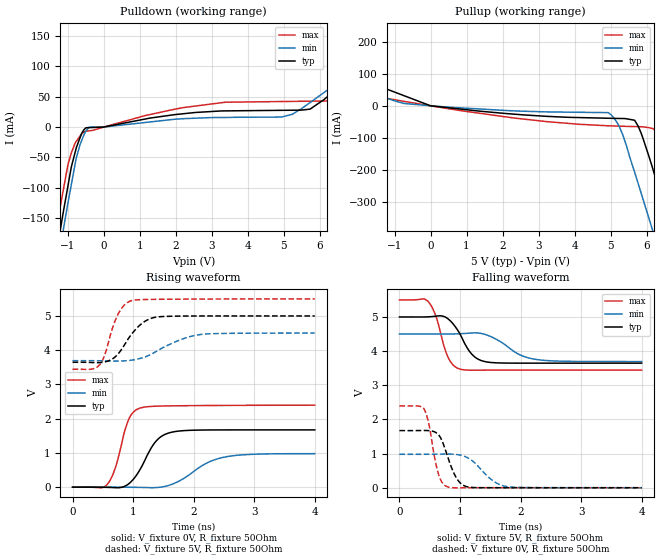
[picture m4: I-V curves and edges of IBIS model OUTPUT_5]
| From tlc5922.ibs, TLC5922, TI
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|   output_5 Model
[Model]   OUTPUT_5
Model_type   Output
Polarity   Non-Inverting
Vmeas = 2.5
Vref = 2.5
Cref = 15pF
Rref = 50
|   typ   min   max
|   (nom PVT)   (Fast PVT)   (slow PVT)
C_comp   1.655e-12   1.559e-12   1.779e-12
|ON state : BUFFER OUTPUT TURNED HIGH
|C_comp   1.655e-12   1.559e-12   1.779e-12
|OFF state: BUFFER OUTPUT TURNED LOW
|C_comp   1.494e-12   1.469e-12   1.521e-12
| Where nom  PVT is Nominal Process,  5V,  65C
|   Fast PVT is Strong Process,   5.5V,  -20C
|   Slow PVT is Weak Process,   4.5V,  125C
[Voltage Range]   5   4.5   5.5
|Ambient Temperature   25   85   -20
|Junction Temperature
[Temperature Range]   65   125   -20
[Pullup Reference]   5   4.5   5.5
[Pulldown Reference]   0   0   0
[Power Clamp Reference]   5   4.5   5.5
[GND Clamp Reference]   0   0   0
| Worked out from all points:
|   slope of the pulldown table from 0 to 0.75 V, typ, clamps not added: 87 ohm
|   slope of the pullup table from 0 to 0.75 V, typ, clamps not added: 81.5 ohm
|   falling waveform, V_fixture 5V, R_fixture 50Ohm: 20-80 % time 276ps typ, 433ps min, 206ps max; typ from 5 V to 3.65 V
|   rising waveform, V_fixture 0V, R_fixture 50Ohm: 20-80 % time 327ps typ, 542ps min, 224ps max; typ from 0 V to 1.67 V
|   rising waveform, V_fixture 5V, R_fixture 50Ohm: 20-80 % time 346ps typ, 567ps min, 233ps max; typ from 3.65 V to 5 V
|   falling waveform, V_fixture 0V, R_fixture 50Ohm: 20-80 % time 213ps typ, 343ps min, 153ps max; typ from 1.67 V to 0 V
[Pulldown]
|   Voltage   I(typ)   I(min)   I(max)
-5V       -1.603A    -1.604A    -1.595A
-1.305V   -205.4mA   -234.4mA   -164.9mA
-1.125V   -141.4mA   -171mA     -105mA
-990.5mV  -96.57mA   -124.8mA   -61.83mA
-755mV    -33.19mA   -49.9mA    -23.03mA
-391mV    -883.4uA   -118.5uA   -6.095mA
2.232V    22.09mA    13.87mA    32.24mA
5.233V    27.75mA    20.88mA    42.27mA
6.44V     61.19mA    70.61mA    47.93mA
8.107V    146.8mA    145mA      144.6mA
8.855V    186.3mA    179.5mA    191.6mA
10V       250.4mA    232.7mA    267.1mA
[Pullup]
|   Voltage   I(typ)   I(min)   I(max)
-5V       213.6mA    187.3mA    242.2mA
-1.188V   50.77mA    22.65mA    22.65mA
0V        0A         0A         0A
4.936V    -38.77mA   -21.32mA   -62.17mA
5.255V    -39.46mA   -67.54mA   -63.38mA
5.665V    -44.88mA   -205.3mA   -64.66mA
5.85V     -85.23mA   -271.8mA   -65.17mA
6.15V     -187.1mA   -380.7mA   -70.24mA
6.473V    -307.6mA   -499.4mA   -112.9mA
6.654V    -374.8mA   -566.2mA   -169mA
7.243V    -596.5mA   -784.5mA   -396mA
10V       -1.65A     -1.818A    -1.473A
[Ramp]
R_load = 50
|   typ   min   max
dV/dt_r   1.00336/3.2663e-10   0.587084/5.42378e-10   1.43592/2.23561e-10
dV/dt_f   0.811682/2.75881e-10   0.483611/4.32773e-10   1.23387/2.05834e-10
[Falling Waveform]
V_fixture = 5V
V_fixture_min = 4.5V
V_fixture_max = 5.5V
R_fixture = 50Ohm
|   Time   V(typ)   V(min)   V(max)
0s        5V         4.5V       5.5V
475ps     5.004V     4.5V       5.453V
600ps     5.023V     4.499V     5.038V
800ps     4.949V     4.5V       3.831V
975ps     4.576V     4.508V     3.487V
1.2ns     3.901V     4.531V     3.442V
1.45ns    3.681V     4.467V     3.443V
1.975ns   3.648V     3.905V     3.444V
2.225ns   3.647V     3.765V     3.444V
4ns       3.647V     3.694V     3.444V
[Rising Waveform]
V_fixture = 0V
V_fixture_min = 0V
V_fixture_max = 0V
R_fixture = 50Ohm
|   Time   V(typ)   V(min)   V(max)
0s        300.2pV    1.699nV    286.7pV
575ps     -6.312mV   794.4uV    84.58mV
700ps     -14.82mV   240.7uV    531.1mV
925ps     93.85mV    -3.088mV   1.972V
1.125ns   547.6mV    -7.671mV   2.316V
1.375ns   1.336V     -12.45mV   2.364V
1.65ns    1.609V     89.18mV    2.375V
2.2ns     1.669V     688mV      2.384V
2.5ns     1.672V     873.9mV    2.387V
4ns       1.672V     978.5mV    2.393V
[Rising Waveform]
V_fixture = 5V
V_fixture_min = 4.5V
V_fixture_max = 5.5V
R_fixture = 50Ohm
|   Time   V(typ)   V(min)   V(max)
0s        3.647V     3.694V     3.443V
325ps     3.64V      3.694V     3.449V
450ps     3.639V     3.691V     3.58V
525ps     3.655V     3.688V     3.829V
650ps     3.736V     3.683V     4.593V
750ps     3.887V     3.682V     5.047V
975ps     4.467V     3.709V     5.447V
1.325ns   4.945V     3.907V     5.484V
2.1ns     4.999V     4.454V     5.493V
4ns       5V         4.5V       5.499V
[Falling Waveform]
V_fixture = 0V
V_fixture_min = 0V
V_fixture_max = 0V
R_fixture = 50Ohm
|   Time   V(typ)   V(min)   V(max)
0s        1.673V     979.2mV    2.395V
400ps     1.676V     979.2mV    2.331V
475ps     1.673V     980mV      1.956V
650ps     1.539V     983.2mV    371mV
800ps     896.2mV    985.8mV    22.48mV
950ps     260.4mV    971.7mV    -3.579mV
1.125ns   24.63mV    878.4mV    -602.5uV
1.55ns    632.5uV    196.2mV    317.7uV
1.775ns   246.1uV    32.81mV    318.1uV
4ns       130.4uV    57.52uV    285.8uV
